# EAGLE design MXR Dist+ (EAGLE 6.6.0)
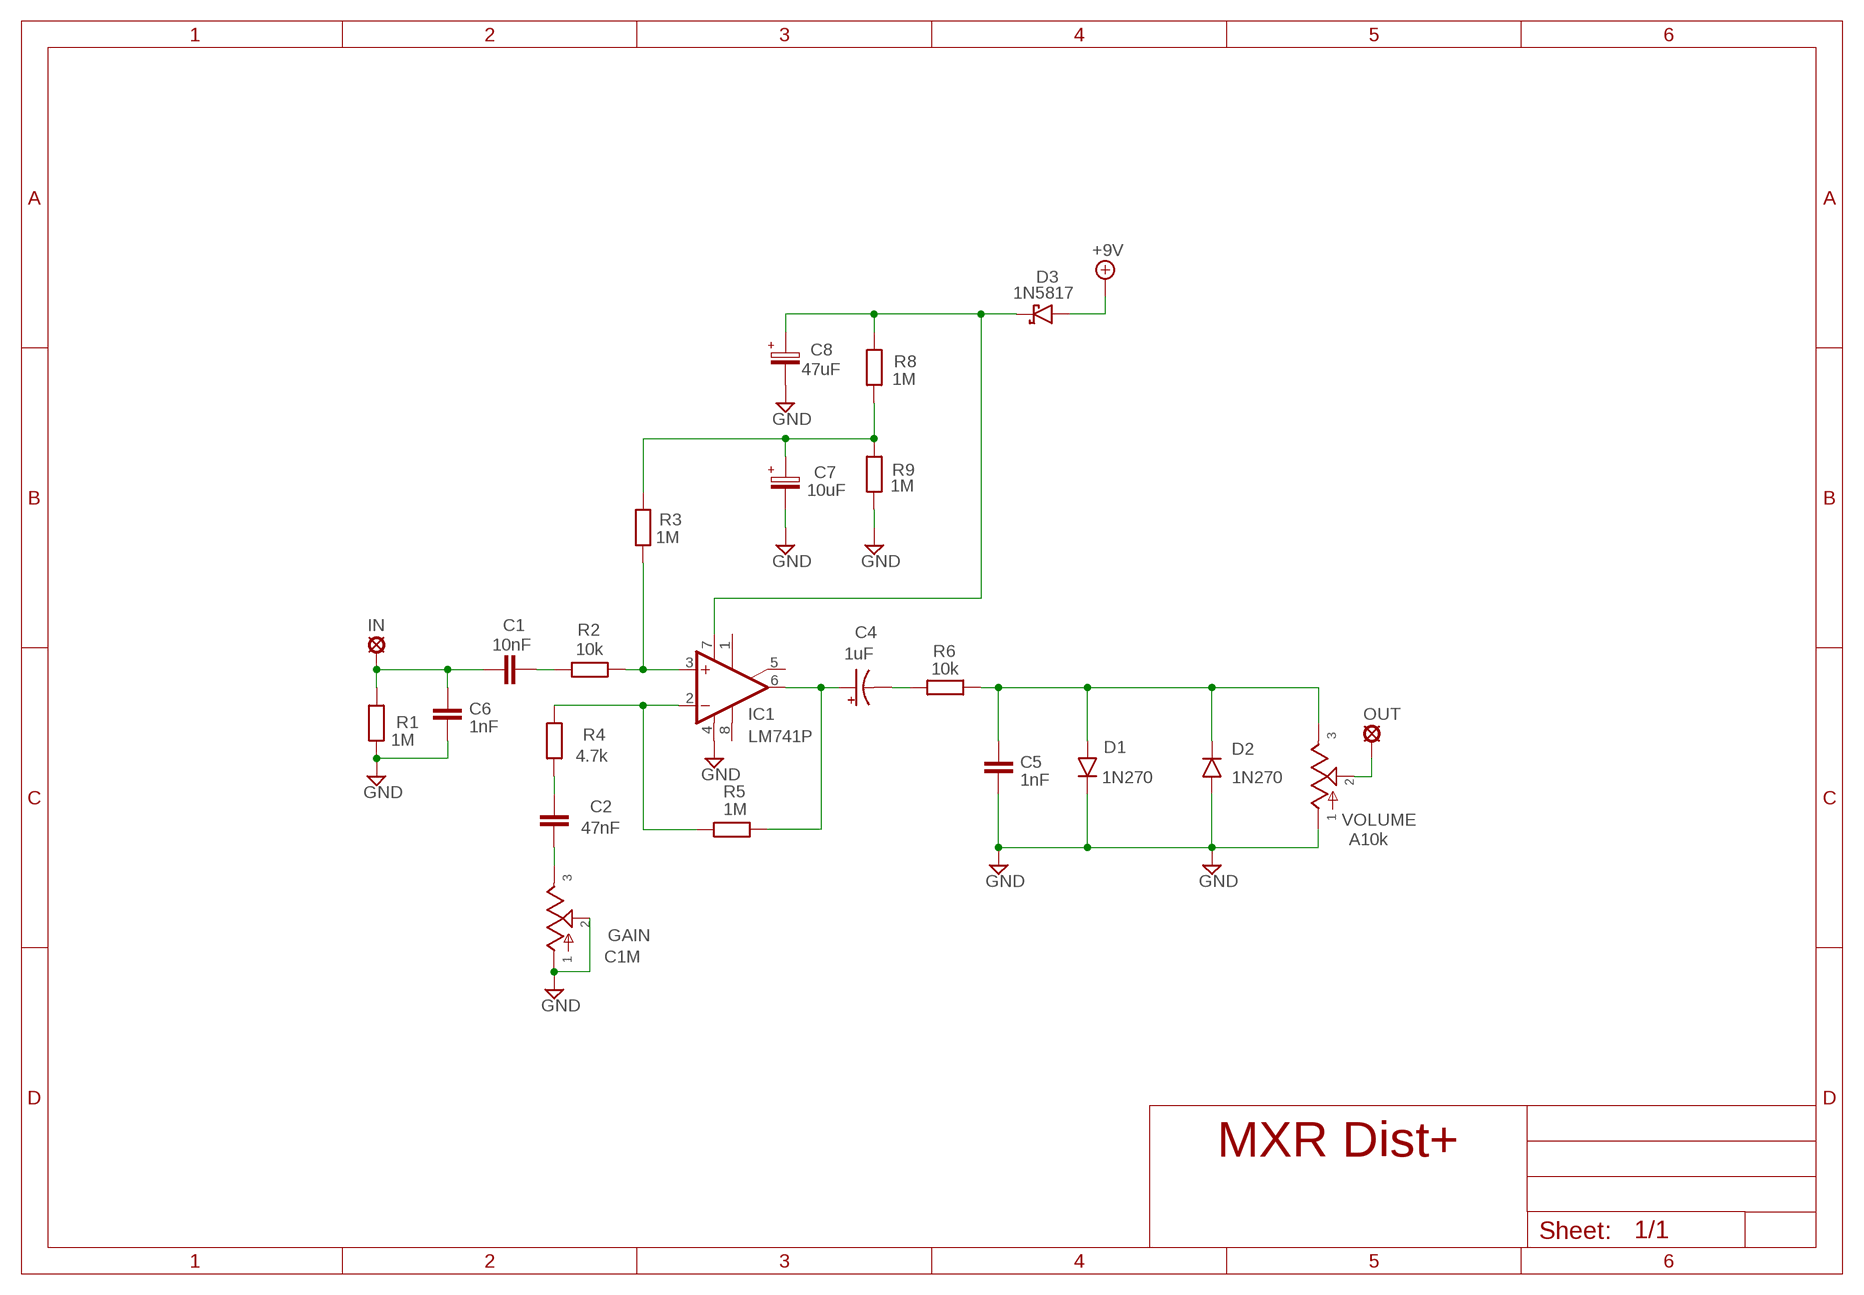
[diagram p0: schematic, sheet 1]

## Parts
+9V  +9V  +9V(T)1  [ROUND]
C1  10nF  1NF-15NF  [3,5MM]
C2  47nF  10NF-47NF"  [4,5MM]
C4  1uF  044A1  [044A]
C5  1nF  1NF-6,8NF  [3,5MM]
C6  1nF  1NF-6,8NF  [3,5MM]
C7  10uF  063-EU  [063_025]
C8  47uF  063-EU  [063_025]
D1  1N270  DO07  [DO07]
D2  1N270  DO07  [DO07]
D3  1N5817  [DO41-3]
GAIN  C1M  POT16MM  [16MM]
GND  GND  GND(T)1  [ROUND]
GND6  GND  GND(T)1  [ROUND]
IC1  LM741P  [DIL08]
IN  MCS10B  [MCS10B]
OUT  MCS10B  [MCS10B]
R1  1M  6MM-EU3  [R0207/3]
R2  10k  6MM-EU3  [R0207/3]
R3  1M  6MM-EU3  [R0207/3]
R4  4.7k  6MM-EU3  [R0207/3]
R5  1M  6MM-EU3  [R0207/3]
R6  10k  6MM-EU3  [R0207/3]
R8  1M  6MM-EU3  [R0207/3]
R9  1M  6MM-EU3  [R0207/3]
VOLUME  A10k  POT16MM  [16MM]

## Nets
+9V: +9V.1(+9V) D3.A
GND: C5.2 C6.2 C7.- C8.- D1.C D2.A GAIN.1 GAIN.2 GND6.1(GND) GND.1(GND) IC1.4(V-) R1.1 R9.1 VOLUME.1
N$1: C2.2 GAIN.3
N$2: C4.2(-) R6.1
N$3: C7.+ R3.2 R8.1 R9.2
N$4: OUT.MP VOLUME.2
N$5: C1.2 R2.1
N$6: IC1.3(+IN) R2.2 R3.1
N$7: C4.1(+) IC1.6(OUT) R5.2
N$8: C5.1 D1.A D2.C R6.2 VOLUME.3
N$9: IC1.2(-IN) R4.2 R5.1
N$10: C2.1 R4.1
N$11: C1.1 C6.1 IN.MP R1.2
N$18: C8.+ D3.C IC1.7(V+) R8.2
Unconnected: IC1.1(ON1) IC1.5(ON2) IC1.8(OPT)

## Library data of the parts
+9V = gm-supply:+9V(T): +9V Voltage Supply
C1 = Mylar Kondensaattorit:1NF-15NF: 1nF-15nF
C2 = Mylar Kondensaattorit:10NF-47NF: 10nF-47nF
C4 = Tantaalit:044A: .1 - 1.5µF
C5 C6 = Mylar Kondensaattorit:1NF-6,8NF: 1nF-6,8nF
C7 C8 = Elektrolyytit:063-EU
D1 D2 = Diodit:DO07: DO-07 Package
D3 = Diodit:1N5817
GAIN VOLUME = gm-pots:POT: Potentiometers the arrow indicates the clockwise motion of th wiper (lug 2) fully counter clockwise there is no resistance between lugs 1 and 2 fully clockwise the resistance between lugs 1 and 2 is the value of the pot
GND GND6 = gm-supply:GND(T): Ground
IC1 = Operaatiovahvistimet:*741: OP AMP
IN OUT = Padit:MCS10B: SOLDER PAD
R1-R6 R8 R9 = Vastukset:6MM-EU: 6mm Resistors (European schematic symbol)

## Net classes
0 default: width 0.406 mm

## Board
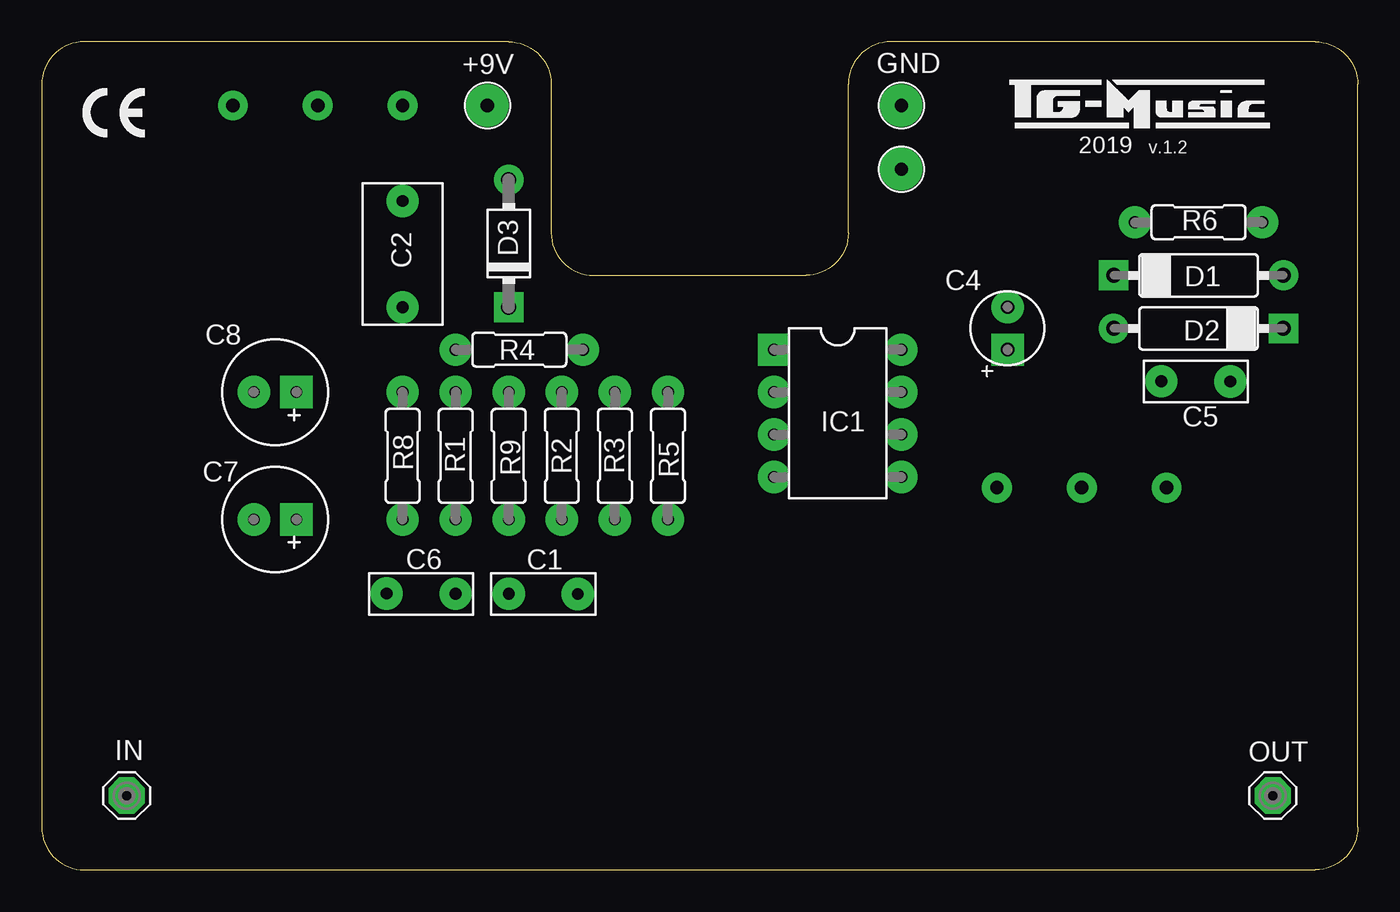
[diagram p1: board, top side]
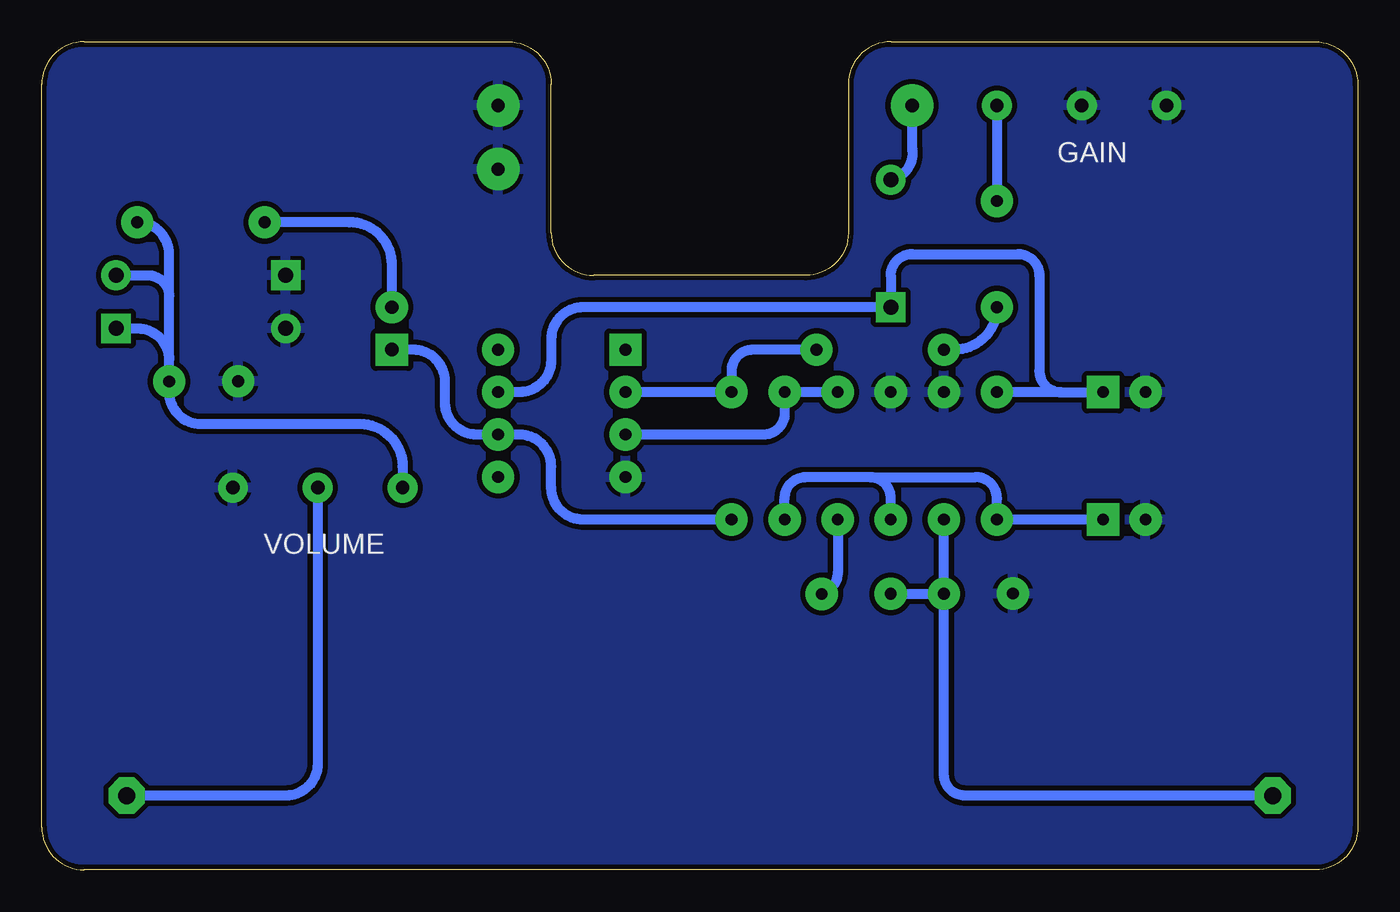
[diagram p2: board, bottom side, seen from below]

Size 78.74 x 49.53 mm. Coordinates in mm from the lower left corner, seen from the top.
Outline: 7.62,49.53 3.81,49.53
Outline: 78.74,2.54 78.74,46.99 arc90 76.2,49.53 50.8,49.53 arc90 48.26,46.99 48.26,38.1 arc-90 45.72,35.56 33.02,35.56 arc-90 30.48,38.1 30.48,46.99 arc90 27.94,49.53 2.54,49.53 arc90 0,46.99 0,2.54 arc90 2.54,0 76.2,0 arc90 78.74,2.54
Copper layers (1*16): Top 0.035mm / dielectric 1.5mm / Bottom 0.035mm
Design rules "ITEADstudio": minimum track width 10mil, minimum drill 12mil, track to track 12mil, track to pad 12mil, pad to pad 12mil, via to via 12mil, smd to smd 0mil, copper to edge 12mil, drill to drill 12mil, minimum pad ring 10mil, minimum via ring 6mil, stop-mask expansion 4mil, vias tented up to drill 100mil, thermal gap 10mil

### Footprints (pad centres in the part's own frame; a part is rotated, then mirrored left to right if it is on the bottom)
ROUND = drill 0.8 pad 2.54: 1 0,0
3,5MM = drill 0.7 pad 1.93: 1 -1.905,0; 2 2.221,-0.016
4,5MM = drill 0.7 pad 1.93: 1 -3.175,0; 2 3.175,0
044A = drill 0.8 pad 1.93 square: 1 -1.27,0 | drill 0.8 pad 1.93: 2 1.27,0
063_025 = drill 0.7 pad 1.93 square: + -1.27,0 | drill 0.7 pad 1.93: - 1.27,0
DO07 = drill 0.9 pad 1.778: A 5.08,0 | drill 0.9 pad 1.778 square: C -5.08,0
DO41-3 = drill 0.9 pad 1.778: A 3.81,0 | drill 0.9 pad 1.778 square: C -3.81,0
16MM = drill 0.8 pad 1.778: 1 5.08,0; 2 0,0; 3 -5.08,0
DIL08 = drill 0.7 pad 1.93 square: 1 -3.81,-3.81 | drill 0.7 pad 1.93: 2 -1.27,-3.81; 3 1.27,-3.81; 4 3.81,-3.81; 5 3.81,3.81; 6 1.27,3.81; 7 -1.27,3.81; 8 -3.81,3.81
MCS10B = drill 1.016 pad 2.159 octagon: MP 0,0
R0207/3 = drill 0.7 pad 1.93: 1 -3.81,0; 2 3.81,0

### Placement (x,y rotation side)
+9V  26.67,45.72 0 top
C1  29.84,16.51 0 top
C2  21.59,36.83 90 top
C4  57.78,32.38 90 top
C5  69.22,29.21 180 top
C6  22.86,16.51 180 top
C7  13.97,20.95 180 top
C8  13.97,28.57 180 top
D1  69.22,35.56 0 top
D2  69.22,32.38 180 top
D3  27.94,37.47 90 top
GAIN  16.51,45.72 180 top
GND  51.44,45.72 0 top
GND6  51.44,41.91 0 top
IC1  47.62,27.3 270 top
IN  5.08,4.45 0 top
OUT  73.66,4.45 0 top
R1  24.77,24.77 270 top
R2  31.11,24.77 90 top
R3  34.29,24.77 270 top
R4  28.57,31.11 0 top
R5  37.47,24.77 270 top
R6  69.22,38.73 0 top
R8  21.59,24.77 90 top
R9  27.94,24.77 270 top
VOLUME  62.23,22.86 0 top

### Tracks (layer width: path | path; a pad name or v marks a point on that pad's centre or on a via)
+9V
  Bottom 0.61: +9V.1 26.67,43.18 arc90 D3.A
GND
  pour Bottom: 0,1.91 0,46.99 arc-90 2.54,49.53 27.94,49.53 arc-90 30.48,46.99 30.48,38.1 arc90 33.02,35.56 45.72,35.56 arc90 48.26,38.1 48.26,46.99 arc-90 50.8,49.53 76.2,49.53 arc-90 78.74,46.99 78.74,2.54 arc-90 76.2,0 1.91,0 arc-90
N$1
  Bottom 0.61: GAIN.3 C2.2
N$2
  Bottom 0.61: C4.2 57.78,36.2 arc-90 60.33,38.73 R6.1
N$3
  Bottom 0.61: R3.2 34.29,22.23 arc90 33.02,23.5 29.21,23.5 | 29.21,23.5 22.86,23.5 arc90 21.59,22.23 R8.1 C7.+ | R9.2 27.94,22.23 arc-90 29.21,23.5
N$4
  Bottom 0.61: VOLUME.2 62.23,6.35 arc90 64.14,4.45 OUT.MP
N$5
  Bottom 0.61: R2.1 31.11,17.78 arc90 32.38,16.51 C1.2
N$6
  Bottom 0.61: R2.2 R3.1 34.29,27.3 arc90 35.56,26.04 IC1.3
N$7
  Bottom 0.61: R5.2 46.35,20.95 arc90 48.26,22.86 48.26,24.13 arc-90 50.16,26.04 IC1.6 52.7,26.04 arc90 54.61,27.94 54.61,29.21 arc-90 56.52,31.11 C4.1
N$8
  Bottom 0.61: VOLUME.3 57.15,24.13 arc-90 59.69,26.67 69.22,26.67 arc90 71.12,28.57 C5.1 71.12,30.48 | 71.12,30.48 71.12,34.29 | 71.12,34.29 71.12,36.83 arc-90 R6.2 | D1.A 72.39,35.56 arc90 71.12,34.29 | D2.C 73.03,32.38 arc90 71.12,30.48
N$9
  Bottom 0.61: R4.2 36.2,31.11 arc-90 37.47,29.84 R5.1 IC1.2
N$10
  Bottom 0.61: C2.1 arc90 24.13,31.11 R4.1
N$11
  Bottom 0.61: C1.1 C6.1 | C6.1 R1.2 | IN.MP 23.5,4.45 arc90 24.77,5.71 C6.1
N$18
  Bottom 0.61: 17.78,28.57 C8.+ | 17.78,28.57 R8.2 | 17.78,28.57 arc90 19.05,29.84 19.05,35.56 arc-90 20.32,36.83 26.67,36.83 arc-90 27.94,35.56 D3.C 46.35,33.66 arc-90 48.26,31.75 48.26,30.48 arc90 50.16,28.57 IC1.7

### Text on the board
tNames: 2019 | v.1.2
tValues: OUT | +9V | GND | IN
